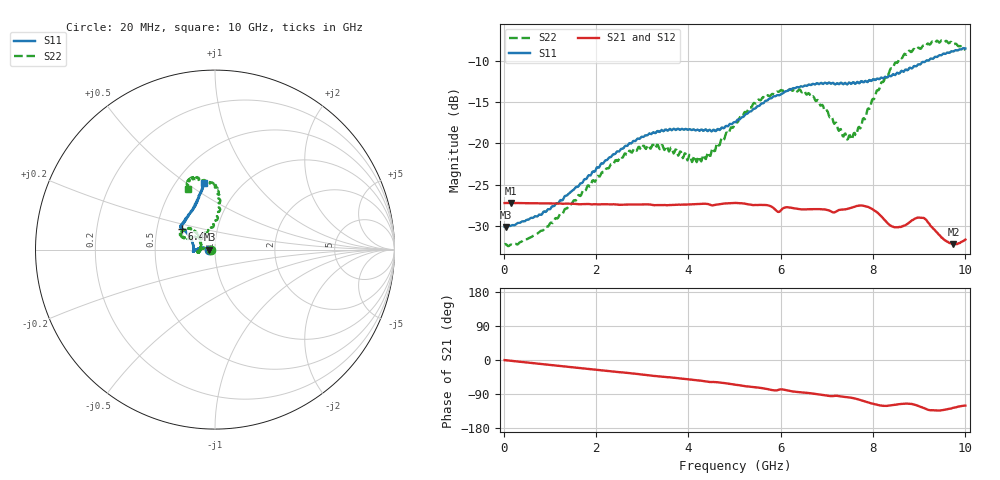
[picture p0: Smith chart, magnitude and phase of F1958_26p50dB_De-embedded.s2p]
! Integrated Device Technology
! Corporate Headquarters
! 6024 Silver Creek Valley Road
! San Jose, CA 95138  USA
! Phone:  1-408-284-8200
! Toll Free:  1-800-223-1366
! Webpage:  http://www.idt.com/
! Timing and RF Division
! 515 Groton Road, Suite 102
! Westford, MA 01886-6024
! Device:  F1958
! Description: 7-bit 0.25 dB Digital Step Attenuator
! Frequency:  0.001 -  6.000 GHz
! Package:  4x4 mm Thin QFN Plastic Package: 24 pin
! Ports:  2 RF, 12 DC
!  Pin  1  = D0
!  Pin  2  = VDD
!  Pin  3  = VMODE
!  Pin  4  = GND
!  Pin  5  = RF1  =  Port 1
!  Pin  6  = GND
!  Pin  7  = GND
!  Pin  8  = GND
!  Pin  9  = GND
!  Pin 10  = GND
!  Pin 11  = GND
!  Pin 12  = GND
!  Pin 13  = GND
!  Pin 14  = RF2  =  Port 2
!  Pin 15  = GND
!  Pin 16  = LE
!  Pin 17  = CLK
!  Pin 18  = DATA
!  Pin 19  = D6
!  Pin 20  = D5
!  Pin 21  = D4
!  Pin 22  = D3
!  Pin 23  = D2
!  Pin 24  = D1
! State:  106
! Atten State:  26.50 dB
! Voltage:  +3.30 Volts
! Current:  0.258 mA
! Data:  The device was measured on a F1958 evaluation board which has
!  individual transmission lines to the RF pins.  Data was collected
!  using a calibrated network analyzer.  The evaluation board was
!  de-embedded using Automatic Fixture Removal (AFR).
!  The reference plane is the edge of the package pin.
! Misc:
!  Action Tracker AT0419
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# GHz S dB R 50
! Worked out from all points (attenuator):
!   500 points, 20 MHz to 10 GHz, reference 50 ohm
!   highest |S21| = -27.24 dB at 160 MHz (marker M1); lowest = -32.3 dB at 9.74 GHz (marker M2)
!   lowest |S11| = -30.2 dB at 40 MHz (marker M3), VSWR 1.06, Z = 47 - j0.045 ohm
!   |S11| at or under -10 dB: start of sweep to 9.14 GHz
!   |S22| runs from -32.5 to -7.5 dB; largest |S21 - S12| = 0.00027
!   S11 on the Smith chart (normalised r, x): 20 MHz: 0.94, -0.00; 6.4 GHz: 0.67, +0.16; 10 GHz: 0.68, +0.59
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0.02  -30.13 -178.9  -27.25 -0.3  -27.24 -0.2  -32.26 -178.9
0.04  -30.15 -179.1  -27.24 -0.5  -27.24 -0.4  -32.23 -178.4
0.16  -30.00 177.6  -27.24 -2.1  -27.24 -2.1  -32.29 178.2
0.84  -28.52 171.2  -27.28 -10.9  -27.28 -10.8  -30.60 172.4
1.7  -24.81 171.2  -27.39 -21.7  -27.38 -21.7  -25.93 171.5
2.62  -20.37 177.2  -27.45 -33.3  -27.42 -33.3  -21.23 -179.3
3.36  -18.59 -175.6  -27.50 -43.1  -27.50 -43.1  -20.50 -169.2
4.24  -18.48 -179.0  -27.37 -54.1  -27.37 -54.2  -21.63 169.1
4.5  -18.54 175.1  -27.53 -58.2  -27.53 -58.2  -20.99 151.5
5.02  -17.41 160.8  -27.24 -65.1  -27.25 -65.1  -17.41 138.2
5.58  -15.16 150.6  -27.48 -73.9  -27.50 -73.9  -14.66 139.9
5.94  -14.13 148.3  -28.32 -79.3  -28.34 -79.3  -13.73 148.7
6.4  -13.18 147.8  -28.00 -84.9  -28.02 -84.8  -13.43 155.9
6.68  -12.82 146.6  -27.99 -88.3  -28.01 -88.2  -14.36 157.9
7.5  -12.65 138.2  -27.89 -99.1  -27.89 -99.1  -19.00 120.0
7.68  -12.60 135.3  -27.57 -103.9  -27.56 -103.8  -18.05 99.8
7.9  -12.41 128.8  -27.74 -112.1  -27.75 -112.1  -15.74 89.4
8.34  -11.79 118.8  -29.82 -120.6  -29.82 -120.7  -11.51 83.9
8.66  -11.31 113.1  -30.01 -115.4  -30.06 -115.5  -9.29 87.7
9.08  -10.09 107.1  -29.05 -126.0  -29.10 -126.1  -8.12 98.9
9.74  -8.83 100.4  -32.27 -126.0  -32.28 -126.4  -7.97 112.0
10  -8.46 99.7  -31.69 -120.4  -31.77 -120.2  -8.65 113.9
